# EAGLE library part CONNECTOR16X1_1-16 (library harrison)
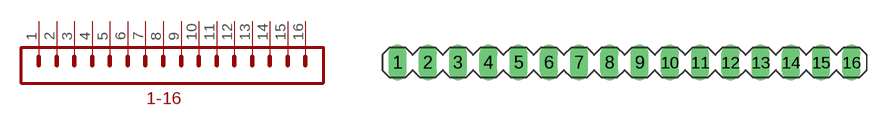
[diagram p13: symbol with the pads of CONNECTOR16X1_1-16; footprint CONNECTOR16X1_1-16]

Designator prefix -

## CONNECTOR16X1_1-16  [CONNECTOR16X1_1-16]
1  P$1  pas
2  P$2  pas
3  P$3  pas
4  P$4  pas
5  P$5  pas
6  P$6  pas
7  P$7  pas
8  P$8  pas
9  P$9  pas
10  P$10  pas
11  P$11  pas
12  P$12  pas
13  P$13  pas
14  P$14  pas
15  P$15  pas
16  P$16  pas

## Footprint CONNECTOR16X1_1-16 (pad centres in mm)
drill 1.016 long: 1 -19.05,0; 2 -16.51,0; 3 -13.97,0; 4 -11.43,0; 5 -8.89,0; 6 -6.35,0; 7 -3.81,0; 8 -1.27,0; 9 1.27,0; 10 3.81,0; 11 6.35,0; 12 8.89,0; 13 11.43,0; 14 13.97,0; 15 16.51,0; 16 19.05,0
